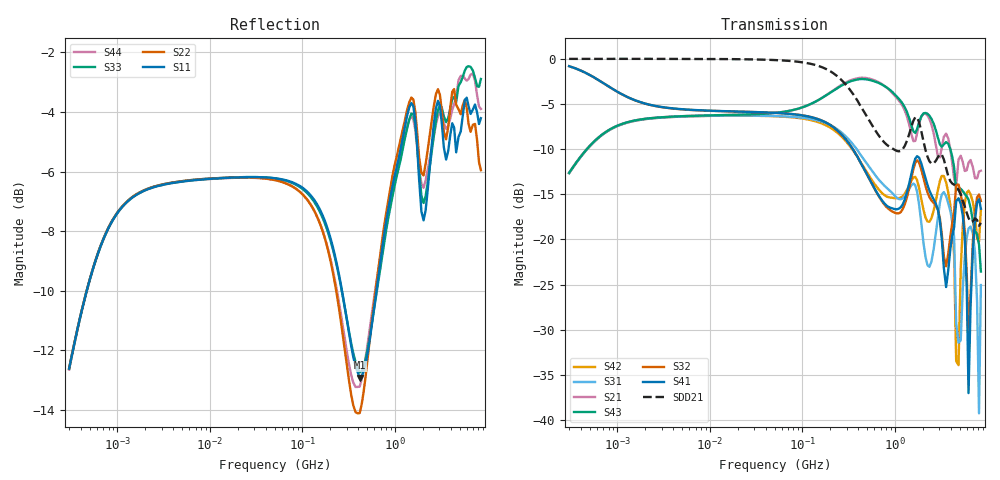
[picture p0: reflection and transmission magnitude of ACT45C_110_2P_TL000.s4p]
! S-Parameter Data Generated by TDK Corporation
! Copyright(C) 2025 TDK Corporation.
! All Rights Reserved.
! TDK P/N: ACT45C-110-2P-TL000 (Signal Line Common Mode Choke/Filter)
! Property: |Zc|=600ohm at 10MHz
! Size(LxWxT): 4.5x3.2x2.8mm
! Model Type: s2p (Touchstone File Format Version 1.0)
! Frequency: DC=Yes Start=0.3MHz Stop=8500MHz 202points Log-sweep
! Model Generated on July 30, 2025
! Terms and conditions regarding TDK Simulation Models:
! 1)This simulation model is being provided solely for informational
!  purposes. Please refer to the specifications of the products in
!  terms of detailed characteristics of such products.
! 2)In no event shall TDK Corporation of any of its subsidiaries be
!  liable for any loss or damage arising, directly or indirectly,
!  from any information contained in this simulation model, including,
!  but not limited to loss or damages arising from any inaccuracies,
!  omissions or errors in connection with such information.
! 3)Any and all copyrights on this simulation model are owned by
!  TDK Corporation.  Duplication or redistribution of this simulation
!  model without prior written permission from TDK Corporation
!  is prohibited.
! 4)This simulation model is subject to any modification or change
!  without any prior notice.
! 5)Neither TDK Corporation nor any of its subsidiaries shall make any
!  warranty, express or implied, including but not limited to the
!  correctness, implied warranties of merchantability and fitness for
!  a particular purpose with respect to this simulation models.
! 6)The use of this simulation model shall be deemed to have consented
!  to the terms and conditions hereof.
! Port Assignments:
!  1 ---@@@--- 4
!  2 ---@@@--- 3
! Applicable Conditions:
!  Temperature = 25 degC
!  DC Bias Current = 0 A
!  Small Signal Operation
# Hz S MA R 50
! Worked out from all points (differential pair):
!   201 points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, 300 kHz to 8.5 GHz, reference 50 ohm
!   strongest paths, dB at 300 kHz, 3.892 MHz, 50.5 MHz, 655.2 MHz, 8.5 GHz:
!     S41: -0.8, -5.5, -6.0, -15.0, -16.6
!     S32: -0.8, -5.5, -6.0, -15.1, -15.8
!     S43: -12.6, -6.4, -6.0, -2.7, -23.6
!     S21: -12.6, -6.4, -6.0, -2.6, -12.4
!     S31: -12.7, -6.5, -6.4, -13.3, -25.0
!     S42: -12.7, -6.5, -6.4, -14.4, -16.7
!   taken as a pair (ports 1,2 in; 4,3 out), SDD21 dB: 0.0, 0.0, -0.2, -8.4, -18.2
!   lowest |S11| = -12.9 dB at 416.2 MHz (marker M1), VSWR 1.58, Z = 79.2 - j0.0882 ohm
!   |S11| at or under -10 dB: start of sweep to 465 kHz; 267.8 MHz to 629.6 MHz (361.8 MHz wide, 80.6 % of centre)
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300000  0.2342 60.3  0.2333 61.3  0.2324 -118.8  0.9077 -13.0
        0.2332 61.3  0.2344 60.3  0.9073 -13.1  0.2323 -118.8
        0.2323 -118.8  0.9077 -13.1  0.234 60.3  0.2331 61.3
        0.9075 -13.0  0.2325 -118.8  0.2333 61.3  0.2333 60.3
4.162441e8  0.226 -0.1  0.7825 -7.6  0.2979 81.7  0.2711 -98.6
            0.7826 -7.6  0.1972 9.8  0.2713 -98.0  0.2721 77.9
            0.298 81.8  0.2711 -97.9  0.2307 -1.1  0.7698 -8.6
            0.271 -98.9  0.2718 77.7  0.77 -8.6  0.2185 7.7
3.378408e9  0.5507 -61.3  0.3689 -56.3  0.1808 15.0  0.07103 -145.9
            0.369 -56.3  0.5848 -59.4  0.08012 -153.0  0.2243 21.2
            0.1825 15.9  0.08087 -151.9  0.6207 -64.9  0.3347 -80.7
            0.06964 -146.5  0.2241 21.1  0.335 -80.8  0.6041 -59.4
4.870722e9  0.5732 -70.3  0.2768 -65.5  0.02669 -149.4  0.1686 -9.8
            0.2768 -65.6  0.6378 -81.1  0.2008 -7.2  0.02022 35.0
            0.02682 -149.3  0.2012 -7.2  0.6982 -80.8  0.1913 -104.6
            0.1688 -10.0  0.02015 33.3  0.1913 -104.7  0.7138 -78.3
6.249568e9  0.6454 -78.7  0.2653 -83.2  0.1159 -17.7  0.01439 -60.4
            0.2655 -83.2  0.6031 -87.4  0.03011 -52.6  0.186 -29.6
            0.1148 -19.0  0.03012 -54.2  0.7533 -90.5  0.1658 -118.5
            0.01412 -62.5  0.1859 -29.7  0.1661 -118.6  0.7166 -87.8
8.115653e9  0.6024 -96.0  0.2371 -110.2  0.01085 -41.5  0.1672 -61.3
            0.2372 -110.3  0.5197 -103.8  0.1777 -69.1  0.09763 -56.6
            0.01091 -41.0  0.1772 -69.3  0.6956 -117.9  0.09355 -140.9
            0.1668 -61.5  0.09731 -56.7  0.09358 -141.0  0.6442 -112.6
8.5e9  0.6161 -98.7  0.2398 -123.8  0.05577 -6.9  0.1477 -87.1
       0.2396 -123.9  0.504 -107.4  0.1625 -92.1  0.1454 -48.2
       0.05591 -7.2  0.1629 -92.1  0.7169 -126.7  0.06632 -156.8
       0.1477 -87.5  0.1458 -48.3  0.06644 -156.9  0.6386 -121.6
